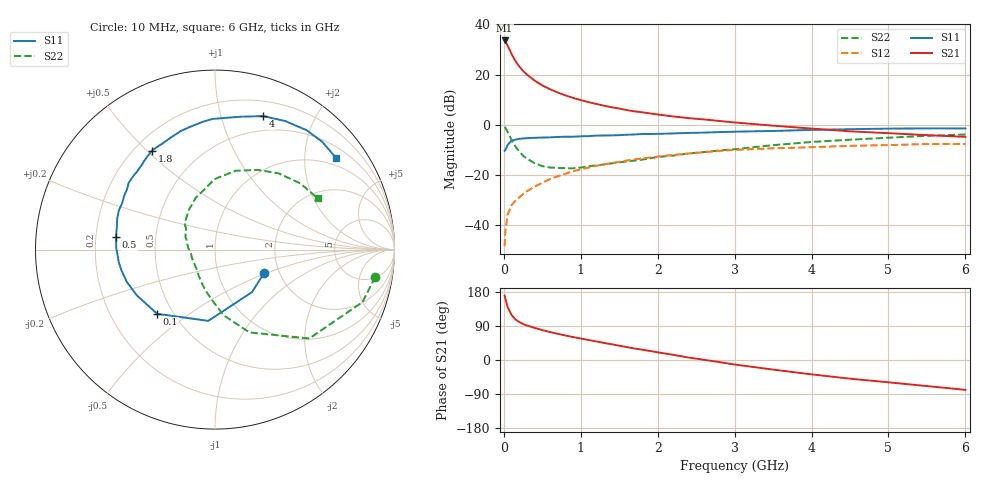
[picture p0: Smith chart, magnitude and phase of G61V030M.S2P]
! SIEMENS Small Signal Semiconductors
! BFG193
! Si NPN RF Bipolar Junction Transistor in SOT223
! VCE = 1 V  IC = 30 mA
! Common Emitter S-Parameters:  August  1996
# GHz  S  MA  R  50
!  f  S11  S21  S12  S22
! GHz  MAG  ANG  MAG  ANG  MAG  ANG  MAG  ANG
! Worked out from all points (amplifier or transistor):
!   36 points, 10 MHz to 6 GHz, reference 50 ohm
!   highest |S21| = 33.6 dB at 10 MHz (marker M1)
!   |S21| within 3 dB of that: start of sweep to 64.04 MHz
!   unconditionally stable (mu >= 1): 449.7 MHz to 2.905 GHz; 3.327 GHz to 3.545 GHz
!   at 250 MHz: K = 0.87, MSG = 24.6 dB, |S12| = -27.6 dB
!   at 1.4 GHz: K = 1.07, MAG = 9.5 dB, |S12| = -15.3 dB
!   at 6 GHz: K = 0.97, MSG = 1.4 dB, |S12| = -7.7 dB
!   S11 on the Smith chart (normalised r, x): 10 MHz: 1.66, -0.48; 100 MHz: 0.41, -0.38; 500 MHz: 0.29, +0.06; 1.8 GHz: 0.27, +0.52; 4 GHz: 0.34, +1.37; 6 GHz: 0.77, +2.78
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0.01  0.3029 -25.7  47.99 170.3  0.0038 83.1  0.9055 -9.7
0.02  0.3142 -48.9  46.05 161.7  0.0076 75.8  0.8722 -19.6
0.05  0.3988 -95.4  37.8 139.3  0.0163 63.9  0.722 -43.3
0.1  0.4815 -132.0  25.86 119.0  0.025 58.2  0.5001 -67.4
0.15  0.5051 -149.8  18.67 107.1  0.0304 56.3  0.3692 -82.5
0.2  0.5235 -160.0  14.61 100.3  0.0356 57.6  0.2929 -91.5
0.25  0.5334 -167.2  11.87 95.0  0.0415 59.0  0.242 -101.1
0.3  0.5405 -172.4  10.02 91.0  0.0472 60.3  0.2124 -108.2
0.4  0.5503 179.1  7.611 84.7  0.0586 61.1  0.1717 -121.9
0.5  0.5564 172.6  6.109 78.8  0.0698 60.7  0.1496 -133.5
0.6  0.5609 167.2  5.12 73.9  0.0825 60.5  0.1406 -143.2
0.8  0.5786 157.7  3.855 64.7  0.1058 57.7  0.1365 -162.2
1.1  0.5934 146.0  2.829 52.8  0.1404 52.4  0.1489 177.2
1.4  0.6144 135.1  2.235 41.6  0.172 45.7  0.17 160.3
1.8  0.6539 122.5  1.773 27.1  0.2134 36.7  0.202 143.3
2.2  0.6718 111.2  1.467 13.7  0.2505 26.7  0.2431 130.2
2.8  0.7146 95.7  1.192 -5.5  0.3014 12.2  0.3075 110.6
3.5  0.7528 79.5  0.96 -25.3  0.3395 -5.5  0.3922 90.5
4  0.7904 70.2  0.84 -37.9  0.3568 -15.1  0.454 75.4
4.5  0.816 61.4  0.741 -49.3  0.3807 -25.0  0.5039 61.8
5.5  0.8471 45.2  0.622 -68.8  0.4138 -47.3  0.6012 37.9
6  0.8459 37.2  0.574 -78.8  0.414 -59.9  0.6406 26.4
